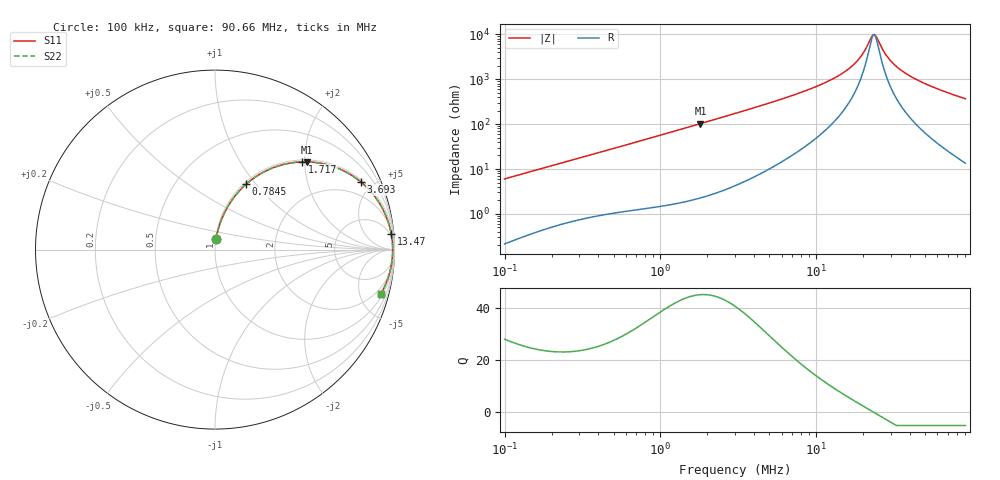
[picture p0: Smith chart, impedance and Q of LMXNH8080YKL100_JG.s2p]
! LMXNH8080YKL100_JG  S-PARAMETER MODEL  ( General Type )
! Model Generated by TAIYO YUDEN Corporation (https://www.yuden.co.jp/en/)
! Version 1.0
! TAIYO YUDEN Control No. 191025NI43SB-FBB
! Copyright(c) 2019 TAIYO YUDEN CO.,LTD. All Rights Reserved.
! Product Description (link to TY-COMPAS)
! https://ds.yuden.co.jp/TYCOMPAS/or/detail?pn=LMXNH8080YKL100MJG&u=M
! Products Name : Inductors
! Characteristics :
!  Inductance : 10 uH , SRF(min) : 22 MHz , DC Resistance(max) : 0.0442 Ohm
!  Rated Current : Saturation :3800 mA , Temp Rise : 3100 mA (40 degC)
!  Case Size : 8.0 x 8.0 / 0.315 x 0.315 [mm/inch] , Thickness : 4 / 0.157 [mm/inch]
!  (Conditions: Temperature = 25 degC , DC Bias Current/Voltage = 0A / 0V)
! External Node Assignments :
!  1  o---GGG---o  2
! GND o---------o GND
! Frequency Range : 0.1MHz  -  90.659724MHz  [ 402 STEP ]
# MHz S RI R 50
! Freq[MHz].  S11 Real  S11 Imag  S21 Real  S21 Imag  S12 Real  S12 Imag  S22 Real  S22 Imag
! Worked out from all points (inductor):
!   401 points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, 100 kHz to 90.66 MHz, reference 50 ohm
!   read as one part in series: L = 9.53 uH near 103.5 kHz
!   highest Q = 45.1 at 1.807 MHz (marker M1), where L = 9.02 uH
!   self-resonance near 23.22 MHz
!   S11 on the Smith chart (normalised r, x): 100 kHz: 1.00, +0.12; 784.5 kHz: 1.03, +0.89; 1.717 MHz: 1.04, +1.94; 3.693 MHz: 1.12, +4.26; 13.47 MHz: 4, +22; 90.66 MHz: 1.27, -7.33
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0.1  0.00574 0.0598  0.9943 -0.0598  0.9943 -0.0598  0.00574 0.0598
0.312872  0.0388 0.1732  0.9612 -0.1732  0.9612 -0.1732  0.0388 0.1732
0.784545  0.1727 0.3637  0.8273 -0.3637  0.8273 -0.3637  0.1727 0.3637
0.97889  0.241 0.4148  0.759 -0.4148  0.759 -0.4148  0.241 0.4148
1.716803  0.4864 0.4888  0.5136 -0.4888  0.5136 -0.4888  0.4864 0.4888
1.806763  0.5116 0.4889  0.4884 -0.4889  0.4884 -0.4889  0.5116 0.4889
3.062674  0.7492 0.4213  0.2508 -0.4213  0.2508 -0.4213  0.7492 0.4213
3.693428  0.8128 0.3766  0.1872 -0.3766  0.1872 -0.3766  0.8128 0.3766
5.652857  0.9107 0.2668  0.0893 -0.2668  0.0893 -0.2668  0.9107 0.2668
9.420503  0.9659 0.1514  0.0341 -0.1514  0.0341 -0.1514  0.9659 0.1514
13.46909  0.9823 0.0861  0.0177 -0.0861  0.0177 -0.0861  0.9823 0.0861
15.96885  0.9865 0.0585  0.0135 -0.0585  0.0135 -0.0585  0.9865 0.0585
18.29877  0.9886 0.0374  0.0114 -0.0374  0.0114 -0.0374  0.9886 0.0374
19.9246  0.9894 0.0245  0.0106 -0.0245  0.0106 -0.0245  0.9894 0.0245
22.44628  0.99 0.00672  0.01 -0.00672  0.01 -0.00672  0.99 0.00672
23.2237  0.99 0.00167  0.00997 -0.00167  0.00997 -0.00167  0.99 0.00167
24.44062  0.99 -0.00591  0.01 0.00591  0.01 0.00591  0.99 -0.00591
27.06907  0.9896 -0.0211  0.0104 0.0211  0.0104 0.0211  0.9896 -0.0211
29.47413  0.9889 -0.034  0.0111 0.034  0.0111 0.034  0.9889 -0.034
34.9443  0.9864 -0.0603  0.0136 0.0603  0.0136 0.0603  0.9864 -0.0603
44.34921  0.9799 -0.0998  0.0201 0.0998  0.0201 0.0998  0.9799 -0.0998
90.65972  0.9228 -0.2491  0.0772 0.2491  0.0772 0.2491  0.9228 -0.2491
